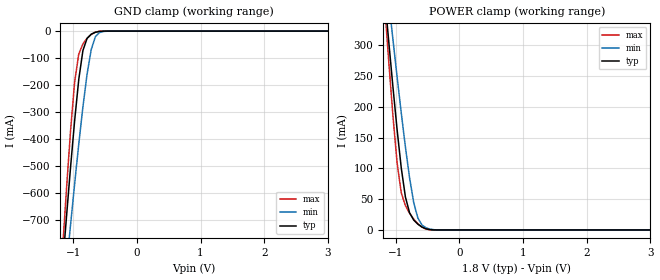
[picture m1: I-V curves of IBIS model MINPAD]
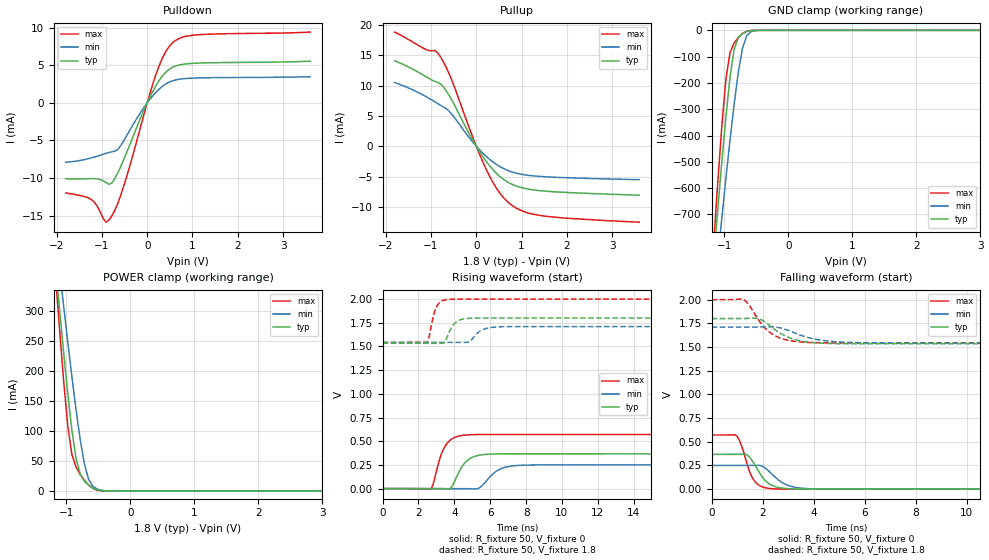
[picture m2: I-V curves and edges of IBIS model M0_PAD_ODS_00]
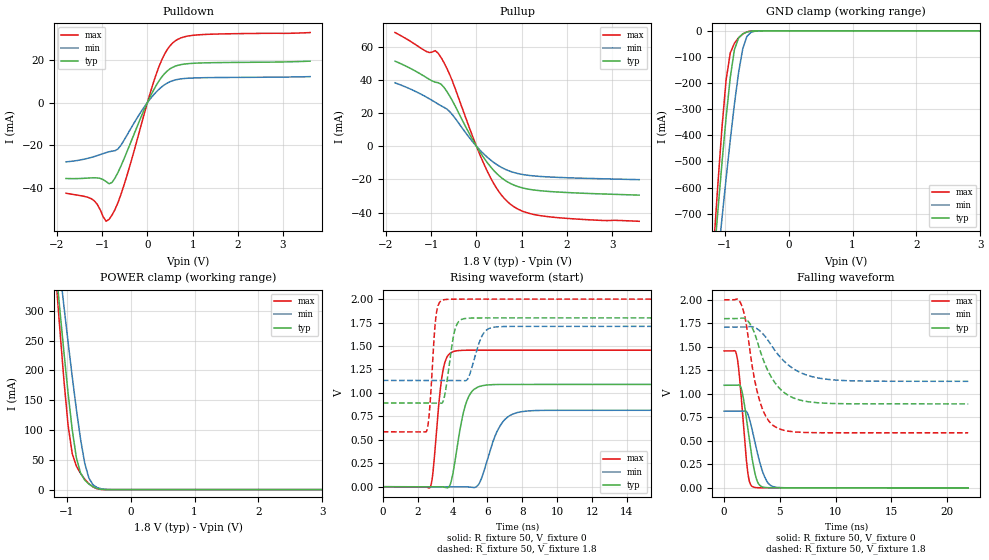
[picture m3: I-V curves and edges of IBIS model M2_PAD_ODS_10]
| Created by SiliconSmart  O-2018.09-SP2-3
[IBIS Ver]   4.0
[File Name]   as34b32bd_1p8_rev1p4.ibs
[File Rev]   1.4
[Date]   Thursday Mar 21 2024
|[Source]   Avalanche Team
|[Notes]   Generated IBIS models from Silicon Smart
|[Rev 1.0]  Initial Release based on extracted netlist
|   Characterization
|[Rev 1.1]  Recharacterization with Hspice, run in high accuracy mode
|[Rev 1.2]  Recharacterization with Hspice, parameters aligned with
|   datasheet
|[Rev 1.3]  Recharacterization with Hspice, run with updated VIH/VIL
|   in parallel with datasheet rev X.7
|[Rev 1.4]  Update the pin to the package pinout assignment
|[Disclaimer]   THE MODEL LIBRARIES ARE PROVIDED AS IS.
|[Copyright]   Copyright 2019, Avalanche Technology., All Rights Reserved
[Component]   AS304GB32_BGA
[Manufacturer] Avalanche Technology
| CONTENT :
| This file contains IBIS MODEL for PSRAM device
| AS304GB32
| USAGE :
| The models are derived for the 1.71V to 2.0V I/O Operation.
| Temperatures for model generation: typ: 25, max: -40, min: 125
| Voltages : typ: 1.8V, min: 1.71V, max: 2.0V
| PACKAGES SUPPORTED :
| 142-ball FBGA (15mm x 17mm)
| VERIFICATION
| Errors  : 0
| Warnings: 11
| All warnings due to non-monotonic data:
[Package]
R_pkg 0   0   0
L_pkg 0   0   0
C_pkg 0   0   0
[Pin]   signal_name   model_name   R_pin   L_pin   C_pin
P8   E#   MINPAD   0.254	7.307E-9	1.178E-12
P7   G#   MINPAD   0.243	7.052E-9	1.094E-12
J2   CR#   MINPAD   0.547	10.386E-9	1.789E-12
K3   PG#   MINPAD   0.451	10.329E-9	1.676E-12
M8   W#   MINPAD   0.377	9.020E-9	1.417E-12
M2   ADDR_26   MINPAD   0.425	9.037E-9	1.604E-12
L4   ADDR_25   MINPAD   0.419	9.644E-9	1.527E-12
K13   ADDR_24   MINPAD   0.495	9.978E-9	1.745E-12
M3   ADDR_23   MINPAD   0.371	9.313E-9	1.466E-12
L3   ADDR_22   MINPAD   0.412	9.753E-9	1.540E-12
M7   ADDR_21   MINPAD   0.368	8.765E-9	1.384E-12
P12   ADDR_20   MINPAD   0.287	8.287E-9	1.639E-12
L12   ADDR_19   MINPAD   0.424	10.320E-9	1.620E-12
N11   ADDR_18   MINPAD   0.338	8.691E-9	1.470E-12
N6   ADDR_17   MINPAD   0.309	8.196E-9	1.279E-12
P6   ADDR_16   MINPAD   0.256	7.462E-9	1.204E-12
L13   ADDR_15   MINPAD   0.463	10.719E-9	1.740E-12
M13   ADDR_14   MINPAD   0.421	10.290E-9	1.689E-12
P10   ADDR_13   MINPAD   0.262	7.671E-9	1.349E-12
N10   ADDR_12   MINPAD   0.340	8.540E-9	1.360E-12
M12   ADDR_11   MINPAD   0.402	9.876E-9	1.604E-12
N13   ADDR_10   MINPAD   0.399	9.819E-9	1.696E-12
L11   ADDR_9   MINPAD   0.443	9.732E-9	1.569E-12
M11   ADDR_8   MINPAD   0.436	9.682E-9	1.671E-12
P5   ADDR_7   MINPAD   0.253	7.464E-9	1.277E-12
P3   ADDR_6   MINPAD   0.279	8.031E-9	1.557E-12
N5   ADDR_5   MINPAD   0.313	8.320E-9	1.359E-12
N4   ADDR_4   MINPAD   0.329	8.138E-9	1.428E-12
M4   ADDR_3   MINPAD   0.379	8.543E-9	1.406E-12
N2   ADDR_2   MINPAD   0.378	9.572E-9	1.637E-12
N9   ADDR_1   MINPAD   0.315	8.416E-9	1.305E-12
M9   ADDR_0   MINPAD   0.403	9.225E-9	1.473E-12
E2   DQ_31   MIOPAD   0.365	8.798E-9	1.454E-12
F2   DQ_30   MIOPAD   0.418	9.057E-9	1.576E-12
D2   DQ_29   MIOPAD   0.358	8.697E-9	1.520E-12
E3   DQ_28   MIOPAD   0.348	8.812E-9	1.441E-12
E12   DQ_27   MIOPAD   0.327	8.506E-9	1.443E-12
D10   DQ_26   MIOPAD   0.309	7.715E-9	1.264E-12
C9   DQ_25   MIOPAD   0.279	7.395E-9	1.219E-12
C7   DQ_24   MIOPAD   0.252	6.802E-9	1.108E-12
G4   DQ_23   MIOPAD   0.455	10.071E-9	1.775E-12
G3   DQ_22   MIOPAD   0.457	10.100E-9	1.750E-12
F13   DQ_21   MIOPAD   0.377	9.387E-9	1.566E-12
D13   DQ_20   MIOPAD   0.295	8.231E-9	1.460E-12
C10   DQ_19   MIOPAD   0.293	7.553E-9	1.298E-12
E8   DQ_18   MIOPAD   0.393	8.323E-9	1.436E-12
F6   DQ_17   MIOPAD   0.425	8.913E-9	1.517E-12
E5   DQ_16   MIOPAD   0.379	8.982E-9	1.460E-12
E13   DQ_15   MIOPAD   0.363	8.555E-9	1.474E-12
G11   DQ_14   MIOPAD   0.475	9.536E-9	1.630E-12
E10   DQ_13   MIOPAD   0.404	8.563E-9	1.453E-12
F9   DQ_12   MIOPAD   0.409	9.347E-9	1.513E-12
C8   DQ_11   MIOPAD   0.257	6.782E-9	1.111E-12
C6   DQ_10   MIOPAD   0.238	7.000E-9	1.114E-12
D6   DQ_9   MIOPAD   0.292	7.776E-9	1.248E-12
D4   DQ_8   MIOPAD   0.305	7.782E-9	1.343E-12
G12   DQ_7   MIOPAD   0.502	10.055E-9	1.687E-12
C12   DQ_6   MIOPAD   0.275	7.857E-9	1.346E-12
D11   DQ_5   MIOPAD   0.286	7.835E-9	1.360E-12
D9   DQ_4   MIOPAD   0.306	8.035E-9	1.299E-12
E7   DQ_3   MIOPAD   0.384	8.178E-9	1.375E-12
C5   DQ_2   MIOPAD   0.231	6.786E-9	1.150E-12
D5   DQ_1   MIOPAD   0.307	7.698E-9	1.346E-12
C3   DQ_0   MIOPAD   0.267	7.420E-9	1.241E-12
G13   INT#   MIOPAD   0.480	10.704E-9	1.759E-12
F10   VSSIO   GND   NA   NA   NA
L10   VSSIO   GND   NA   NA   NA
E9   VSSIO   GND   NA   NA   NA
L9   VSSIO   GND   NA   NA   NA
F8   VSSIO   GND   NA   NA   NA
L8   VSSIO   GND   NA   NA   NA
F7   VSSIO   GND   NA   NA   NA
L7   VSSIO   GND   NA   NA   NA
E6   VSSIO   GND   NA   NA   NA
L6   VSSIO   GND   NA   NA   NA
G5   VSSIO   GND   NA   NA   NA
A14   VSS   GND   NA   NA   NA
B14   VSS   GND   NA   NA   NA
C14   VSS   GND   NA   NA   NA
H13   VSS   GND   NA   NA   NA
R14   VSS   GND   NA   NA   NA
T14   VSS   GND   NA   NA   NA
A13   VSS   GND   NA   NA   NA
T13   VSS   GND   NA   NA   NA
A12   VSS   GND   NA   NA   NA
G10   VSS   GND   NA   NA   NA
H10   VSS   GND   NA   NA   NA
J10   VSS   GND   NA   NA   NA
K10   VSS   GND   NA   NA   NA
F5   VSS   GND   NA   NA   NA
L5   VSS   GND   NA   NA   NA
A2   VSS   GND   NA   NA   NA
T2   VSS   GND   NA   NA   NA
A1   VSS   GND   NA   NA   NA
B1   VSS   GND   NA   NA   NA
R1   VSS   GND   NA   NA   NA
T1   VSS   GND   NA   NA   NA
F12   VCCIO   POWER   NA   NA   NA
J12   VCCIO   POWER   NA   NA   NA
E11   VCCIO   POWER   NA   NA   NA
M10   VCCIO   POWER   NA   NA   NA
D8   VCCIO   POWER   NA   NA   NA
N8   VCCIO   POWER   NA   NA   NA
D7   VCCIO   POWER   NA   NA   NA
N7   VCCIO   POWER   NA   NA   NA
M5   VCCIO   POWER   NA   NA   NA
E4   VCCIO   POWER   NA   NA   NA
F3   VCCIO   POWER   NA   NA   NA
J3   VCCIO   POWER   NA   NA   NA
C13   VCC   POWER   NA   NA   NA
P13   VCC   POWER   NA   NA   NA
D12   VCC   POWER   NA   NA   NA
N12   VCC   POWER   NA   NA   NA
C11   VCC   POWER   NA   NA   NA
F11   VCC   POWER   NA   NA   NA
H11   VCC   POWER   NA   NA   NA
J11   VCC   POWER   NA   NA   NA
K11   VCC   POWER   NA   NA   NA
P11   VCC   POWER   NA   NA   NA
C4   VCC   POWER   NA   NA   NA
F4   VCC   POWER   NA   NA   NA
H4   VCC   POWER   NA   NA   NA
J4   VCC   POWER   NA   NA   NA
K4   VCC   POWER   NA   NA   NA
P4   VCC   POWER   NA   NA   NA
D3   VCC   POWER   NA   NA   NA
N3   VCC   POWER   NA   NA   NA
C2   VCC   POWER   NA   NA   NA
P2   VCC   POWER   NA   NA   NA
|[Package Model]   Package model name.  40-char limit.
|   (fill in and uncomment to use this section)
| IOPAD
[Model Selector] MIOPAD
| Model Description
M0_PAD_ODS_00   ODS_00
M1_PAD_ODS_01   ODS_01
M2_PAD_ODS_10   ODS_10
M3_PAD_ODS_11   ODS_11
| Models and submodels in the file (5): MINPAD (Input), M0_PAD_ODS_00 (I/O), M2_PAD_ODS_10 (I/O), M1_PAD_ODS_01 (I/O), M3_PAD_ODS_11 (I/O)
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[Model] MINPAD
Model_type Input
Enable   Active-High
Vinl  =  0.63
Vinh  =  1.17
| Capacitance  typ   min   max
C_comp   6.497054e-12   6.073083e-12   6.958902e-12
| Variables   typ   min   max
[GND Clamp Reference]   0   0   0
[POWER Clamp Reference]   1.8   1.71   2
[Pulldown Reference]   0   0   0
[Pullup Reference]   1.8   1.71   2
[Temperature Range]   25   125   -40
[Voltage Range]   1.8   1.71   2
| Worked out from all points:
|   GND clamp passes 1 mA (typ) near -0.58 V on its own axis
|   POWER clamp passes 1 mA (typ) near -0.48 V on its own axis
[GND Clamp]
| Voltage   I(typ)   I(min)   I(max)
-1.8V     -2.882A    -2.682A    -3.302A
-1.173V   -889.3mA   -1.041A    -830.7mA
-1.108V   -695.2mA   -879.1mA   -594mA
-1.043V   -507.9mA   -720.4mA   -373.1mA
-977.6mV  -332.2mA   -566.2mA   -188.7mA
-912.4mV  -178.9mA   -418.3mA   -84.89mA
-847.2mV  -71.94mA   -280.4mA   -47.65mA
-782.1mV  -27.06mA   -159.4mA   -26.6mA
-716.9mV  -11.75mA   -68.54mA   -12.18mA
-651.7mV  -4.473mA   -21mA      -3.799mA
-456.2mV  -15.9uA    -297.6uA   -1.679uA
3.6V      0A         0A         0A
[POWER Clamp]
| Voltage   I(typ)   I(min)   I(max)
-1.8V     1.148A     1.073A     1.318A
-1.173V   379.5mA    433.8mA    364.1mA
-1.108V   304.4mA    370.6mA    271.9mA
-1.043V   231.6mA    308.7mA    184.6mA
-977.6mV  162.5mA    248.2mA    108.6mA
-912.4mV  100.5mA    189.8mA    60.25mA
-847.2mV  53.5mA     134.6mA    39.41mA
-716.9mV  16.06mA    44.37mA    17.57mA
-651.7mV  9.361mA    19.28mA    9.931mA
-586.6mV  4.721mA    8.013mA    4.451mA
-325.9mV  4.613uA    79.39uA    440.6nA
3.6V      0A         0A         0A
[Model] M0_PAD_ODS_00
Model_type I/O
Enable   Active-High
Vinl  =  0.63
Vinh  =  1.17
Vmeas =  0.9
Cref  =  30e-12
| Capacitance  typ   min   max
C_comp   6.492186e-12   6.071794e-12   6.967131e-12
| Variables   typ   min   max
[GND Clamp Reference]   0   0   0
[POWER Clamp Reference]   1.8   1.71   2
[Pulldown Reference]   0   0   0
[Pullup Reference]   1.8   1.71   2
[Temperature Range]   25   125   -40
[Voltage Range]   1.8   1.71   2
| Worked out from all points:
|   slope of the pulldown table from 0 to 0.27 V, typ, clamps not added: 89.8 ohm
|   slope of the pullup table from 0 to 0.27 V, typ, clamps not added: 90.4 ohm
|   GND clamp passes 1 mA (typ) near -0.58 V on its own axis
|   POWER clamp passes 1 mA (typ) near -0.48 V on its own axis
|   falling waveform, R_fixture 50, V_fixture 0: 20-80 % time 567ps typ, 700ps min, 438ps max; typ from 0.367 V to 0 V
|   falling waveform, R_fixture 50, V_fixture 1.8: 20-80 % time 987ps typ, 1.2ns min, 841ps max; typ from 1.8 V to 1.53 V
|   rising waveform, R_fixture 50, V_fixture 0: 20-80 % time 695ps typ, 848ps min, 610ps max; typ from 0 V to 0.367 V
|   rising waveform, R_fixture 50, V_fixture 1.8: 20-80 % time 469ps typ, 591ps min, 352ps max; typ from 1.53 V to 1.8 V
[GND Clamp]
| Voltage   I(typ)   I(min)   I(max)
-1.8V     -2.882A    -2.682A    -3.302A
-1.173V   -889.3mA   -1.041A    -830.7mA
-1.108V   -695.2mA   -879.1mA   -594mA
-1.043V   -507.9mA   -720.4mA   -373.2mA
-977.6mV  -332.2mA   -566.2mA   -188.7mA
-912.4mV  -178.9mA   -418.3mA   -84.9mA
-847.2mV  -71.94mA   -280.4mA   -47.66mA
-782.1mV  -27.06mA   -159.4mA   -26.61mA
-716.9mV  -11.75mA   -68.54mA   -12.18mA
-651.7mV  -4.473mA   -21mA      -3.801mA
-456.2mV  -15.91uA   -297.6uA   -1.681uA
3.6V      0A         0A         0A
[POWER Clamp]
| Voltage   I(typ)   I(min)   I(max)
-1.8V     1.148A     1.073A     1.318A
-1.173V   379.5mA    433.8mA    364.1mA
-1.108V   304.4mA    370.6mA    271.9mA
-1.043V   231.6mA    308.7mA    184.6mA
-977.6mV  162.5mA    248.2mA    108.6mA
-912.4mV  100.5mA    189.8mA    60.25mA
-847.2mV  53.5mA     134.6mA    39.41mA
-716.9mV  16.06mA    44.37mA    17.57mA
-651.7mV  9.361mA    19.28mA    9.931mA
-586.6mV  4.721mA    8.013mA    4.451mA
-325.9mV  4.613uA    79.39uA    440.6nA
3.6V      0A         0A         0A
[Pulldown]
| Voltage   I(typ)   I(min)   I(max)
-1.8V     -10.09mA   -7.898mA   -11.97mA
-1.238V   -10.07mA   -7.33mA    -12.83mA
-912.4mV  -10.59mA   -6.717mA   -15.86mA
-847.2mV  -10.83mA   -6.605mA   -15.6mA
-716.9mV  -10.08mA   -6.431mA   -14.3mA
-521.4mV  -7.575mA   -5.077mA   -11.12mA
-65.17mV  -872uA     -545.4uA   -1.404mA
248.3mV   2.817mA    1.73mA     4.683mA
434.5mV   4.193mA    2.586mA    7.041mA
620.7mV   4.869mA    3.026mA    8.258mA
1.179V    5.284mA    3.307mA    9.058mA
3.6V      5.531mA    3.462mA    9.391mA
[Pullup]
| Voltage   I(typ)   I(min)   I(max)
-1.8V     14.07mA    10.49mA    18.8mA
-1.108V   11.45mA    8.161mA    15.93mA
-912.4mV  10.66mA    7.301mA    15.78mA
-782.1mV  10.22mA    6.706mA    14.62mA
-586.6mV  8.214mA    5.673mA    11.74mA
-65.17mV  835.7uA    571.5uA    1.251mA
248.3mV   -2.782mA   -1.866mA   -4.251mA
496.6mV   -4.831mA   -3.242mA   -7.473mA
744.8mV   -6.111mA   -4.126mA   -9.499mA
1.055V    -6.927mA   -4.698mA   -10.78mA
1.428V    -7.337mA   -4.986mA   -11.42mA
3.6V      -8.069mA   -5.52mA    -12.52mA
[Ramp]
dV/dt_r   0.220223/0.695182n  0.150081/0.847662n  0.34276/0.610066n
dV/dt_f   0.159898/0.986852n  0.100157/1.19933n  0.274317/0.841199n
R_load = 50
[Falling Waveform]
R_fixture = 50
V_fixture = 0
V_fixture_min = 0
V_fixture_max = 0
| Time   V(typ)   V(min)   V(max)
0s        367mV      250.1mV    571.3mV
970.5ps   367.6mV    250.7mV    565.8mV
1.163ns   367.7mV    250.8mV    465.6mV
1.366ns   364.8mV    250.9mV    289.2mV
1.633ns   283.2mV    251.1mV    104.5mV
1.912ns   159.1mV    248.9mV    32.86mV
2.259ns   56.6mV     186.1mV    7.625mV
2.939ns   6.435mV    44.81mV    470.9uV
3.847ns   401uV      4.515mV    161.3uV
21.88ns   789.3nV    339.8nV    -894.6nV
[Falling Waveform]
R_fixture = 50
V_fixture = 1.8
V_fixture_min = 1.71
V_fixture_max = 2
| Time   V(typ)   V(min)   V(max)
0s        1.8V       1.71V      2V
1.279ns   1.801V     1.71V      1.996V
1.474ns   1.804V     1.711V     1.942V
1.822ns   1.8V       1.711V     1.793V
2.315ns   1.719V     1.713V     1.648V
2.827ns   1.625V     1.692V     1.583V
3.341ns   1.573V     1.64V      1.556V
4.254ns   1.542V     1.574V     1.545V
5.785ns   1.534V     1.546V     1.543V
21.88ns   1.534V     1.543V     1.543V
[Rising Waveform]
R_fixture = 50
V_fixture = 0
V_fixture_min = 0
V_fixture_max = 0
| Time   V(typ)   V(min)   V(max)
0s        8.086nV    337.8nV    6.906nV
2.695ns   -605.3uV   -543.5uV   -2.704mV
3.178ns   -713.5uV   -640.8uV   307mV
3.478ns   -2.128mV   -701.4uV   444.8mV
3.826ns   11.64mV    -771.6uV   519.1mV
4.54ns    260.3mV    -915.7uV   563.8mV
5.312ns   348.7mV    -240.6uV   570.4mV
6.469ns   365.9mV    197.8mV    570.4mV
7.493ns   366.4mV    244mV      570.5mV
21.88ns   367mV      250.1mV    571.3mV
[Rising Waveform]
R_fixture = 50
V_fixture = 1.8
V_fixture_min = 1.71
V_fixture_max = 2
| Time   V(typ)   V(min)   V(max)
0s        1.534V     1.543V     1.543V
2.471ns   1.533V     1.543V     1.544V
2.994ns   1.533V     1.543V     1.912V
3.427ns   1.538V     1.543V     1.989V
3.704ns   1.646V     1.543V     1.997V
4.14ns    1.762V     1.543V     2V
4.864ns   1.797V     1.553V     2V
5.531ns   1.8V       1.672V     2V
6.499ns   1.8V       1.707V     2V
21.88ns   1.8V       1.71V      2V
[Model] M2_PAD_ODS_10
Model_type I/O
Enable   Active-High
Vinl  =  0.63
Vinh  =  1.17
Vmeas =  0.9
Cref  =  30e-12
| Capacitance  typ   min   max
C_comp   6.492186e-12   6.071794e-12   6.967131e-12
| Variables   typ   min   max
[GND Clamp Reference]   0   0   0
[POWER Clamp Reference]   1.8   1.71   2
[Pulldown Reference]   0   0   0
[Pullup Reference]   1.8   1.71   2
[Temperature Range]   25   125   -40
[Voltage Range]   1.8   1.71   2
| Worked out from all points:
|   slope of the pulldown table from 0 to 0.27 V, typ, clamps not added: 25.7 ohm
|   slope of the pullup table from 0 to 0.27 V, typ, clamps not added: 24.7 ohm
|   GND clamp passes 1 mA (typ) near -0.58 V on its own axis
|   POWER clamp passes 1 mA (typ) near -0.48 V on its own axis
|   falling waveform, R_fixture 50, V_fixture 0: 20-80 % time 814ps typ, 1.03ns min, 609ps max; typ from 1.09 V to 0 V
|   falling waveform, R_fixture 50, V_fixture 1.8: 20-80 % time 2.03ns typ, 2.69ns min, 1.33ns max; typ from 1.8 V to 0.893 V
|   rising waveform, R_fixture 50, V_fixture 0: 20-80 % time 649ps typ, 942ps min, 438ps max; typ from 0 V to 1.09 V
|   rising waveform, R_fixture 50, V_fixture 1.8: 20-80 % time 428ps typ, 581ps min, 290ps max; typ from 0.893 V to 1.8 V
[GND Clamp]
| Voltage   I(typ)   I(min)   I(max)
-1.8V     -2.882A    -2.682A    -3.302A
-1.173V   -889.3mA   -1.041A    -830.7mA
-1.108V   -695.2mA   -879.1mA   -594mA
-1.043V   -507.9mA   -720.4mA   -373.2mA
-977.6mV  -332.2mA   -566.2mA   -188.7mA
-912.4mV  -178.9mA   -418.3mA   -84.9mA
-847.2mV  -71.94mA   -280.4mA   -47.66mA
-782.1mV  -27.06mA   -159.4mA   -26.61mA
-716.9mV  -11.75mA   -68.54mA   -12.18mA
-651.7mV  -4.473mA   -21mA      -3.801mA
-456.2mV  -15.91uA   -297.6uA   -1.681uA
3.6V      0A         0A         0A
[POWER Clamp]
| Voltage   I(typ)   I(min)   I(max)
-1.8V     1.148A     1.073A     1.318A
-1.173V   379.5mA    433.8mA    364.1mA
-1.108V   304.4mA    370.6mA    271.9mA
-1.043V   231.6mA    308.7mA    184.6mA
-977.6mV  162.5mA    248.2mA    108.6mA
-912.4mV  100.5mA    189.8mA    60.25mA
-847.2mV  53.5mA     134.6mA    39.41mA
-716.9mV  16.06mA    44.37mA    17.57mA
-651.7mV  9.361mA    19.28mA    9.931mA
-586.6mV  4.721mA    8.013mA    4.451mA
-325.9mV  4.613uA    79.39uA    440.6nA
3.6V      0A         0A         0A
[Pulldown]
| Voltage   I(typ)   I(min)   I(max)
-1.8V     -35.45mA   -27.68mA   -42.34mA
-1.238V   -35.17mA   -25.59mA   -44.93mA
-912.4mV  -36.92mA   -23.37mA   -55.44mA
-847.2mV  -37.89mA   -22.97mA   -54.5mA
-716.9mV  -35.26mA   -22.46mA   -49.94mA
-521.4mV  -26.49mA   -17.75mA   -38.78mA
-65.17mV  -3.048mA   -1.907mA   -4.891mA
248.3mV   9.844mA    6.047mA    16.33mA
434.5mV   14.66mA    9.037mA    24.58mA
620.7mV   17.01mA    10.57mA    28.86mA
1.179V    18.47mA    11.56mA    31.67mA
3.6V      19.32mA    12.09mA    32.66mA
[Pullup]
| Voltage   I(typ)   I(min)   I(max)
-1.8V     51.26mA    38.2mA     68.51mA
-1.108V   41.41mA    29.63mA    57.12mA
-912.4mV  38.62mA    26.49mA    57.6mA
-782.1mV  37.38mA    24.37mA    53.47mA
-586.6mV  30.05mA    20.74mA    42.91mA
-65.17mV  3.056mA    2.089mA    4.574mA
248.3mV   -10.17mA   -6.821mA   -15.55mA
496.6mV   -17.67mA   -11.85mA   -27.35mA
744.8mV   -22.35mA   -15.08mA   -34.79mA
1.055V    -25.34mA   -17.17mA   -39.5mA
1.49V     -26.99mA   -18.33mA   -42.12mA
3.6V      -29.47mA   -20.13mA   -45.23mA
[Ramp]
dV/dt_r   0.654716/0.649264n  0.489281/0.942172n  0.873692/0.437773n
dV/dt_f   0.544072/2.0345n  0.346027/2.68971n  0.848874/1.32832n
R_load = 50
[Falling Waveform]
R_fixture = 50
V_fixture = 0
V_fixture_min = 0
V_fixture_max = 0
| Time   V(typ)   V(min)   V(max)
0s        1.091V     815.5mV    1.456V
1.134ns   1.092V     815.8mV    1.408V
1.355ns   1.095V     815.9mV    1.215V
1.576ns   1.041V     815.9mV    909.4mV
2.09ns    659.1mV    795.4mV    194.4mV
2.556ns   281.2mV    596.9mV    11.89mV
3.162ns   31.14mV    287.7mV    1.067mV
3.764ns   3.174mV    83.95mV    957.3uV
4.408ns   740.4uV    12.61mV    923.2uV
21.88ns   -295.3nV   254.4nV    -62.01nV
[Falling Waveform]
R_fixture = 50
V_fixture = 1.8
V_fixture_min = 1.71
V_fixture_max = 2
| Time   V(typ)   V(min)   V(max)
0s        1.8V       1.71V      2V
1.528ns   1.806V     1.711V     1.955V
1.972ns   1.793V     1.712V     1.753V
2.371ns   1.736V     1.716V     1.41V
3.153ns   1.488V     1.675V     940.7mV
3.743ns   1.295V     1.601V     759.2mV
4.802ns   1.081V     1.423V     634.2mV
6.39ns    948.9mV    1.254V     594.4mV
8.536ns   903.6mV    1.166V     586.3mV
21.88ns   893.2mV    1.133V     585.2mV
[Rising Waveform]
R_fixture = 50
V_fixture = 0
V_fixture_min = 0
V_fixture_max = 0
| Time   V(typ)   V(min)   V(max)
0s        4.211nV    196.7nV    3.157nV
2.711ns   -419.1uV   -333uV     -6.987mV
2.878ns   -445uV     -353.6uV   156.9mV
3.41ns    -1.187mV   -419uV     1.198V
4.002ns   124.7mV    -491.8uV   1.439V
4.74ns    872.2mV    -582.4uV   1.455V
5.668ns   1.076V     93.9mV     1.456V
6.722ns   1.09V      648.9mV    1.456V
7.703ns   1.09V      790.3mV    1.456V
21.88ns   1.091V     815.5mV    1.456V
[Rising Waveform]
R_fixture = 50
V_fixture = 1.8
V_fixture_min = 1.71
V_fixture_max = 2
| Time   V(typ)   V(min)   V(max)
0s        893.2mV    1.133V     585.2mV
2.514ns   892.5mV    1.133V     595.7mV
2.696ns   892.4mV    1.133V     855.6mV
3.056ns   892.3mV    1.133V     1.83V
3.446ns   905.1mV    1.133V     1.991V
4.094ns   1.642V     1.132V     2V
4.629ns   1.791V     1.132V     2V
5.714ns   1.8V       1.617V     2V
6.323ns   1.8V       1.699V     2V
21.88ns   1.8V       1.71V      2V
